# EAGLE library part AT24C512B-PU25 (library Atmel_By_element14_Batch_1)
Two-wire Serial EEPROM
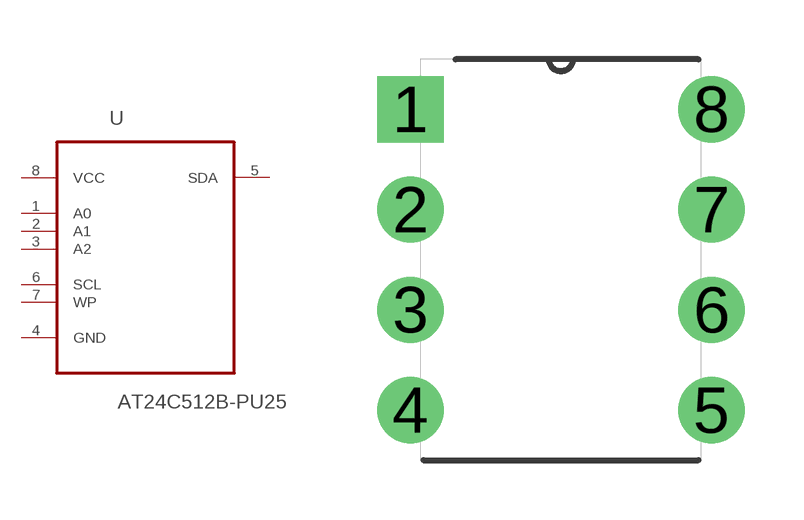
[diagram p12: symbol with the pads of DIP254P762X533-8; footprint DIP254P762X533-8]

Designator prefix U

## AT24C512B-PU25 (MPN: AT24C512B-PU25; OC_FARNELL: 1362655; OC_NEWARK: -; PACKAGE: PDIP-8; SUPPLIER: Atmel)  [DIP254P762X533-8]
1  A0  in
2  A1  in
3  A2  in
4  GND  pas
5  SDA
6  SCL  in
7  WP  pas
8  VCC  pwr

## Footprint DIP254P762X533-8 (pad centres in mm)
drill 1.118 square: 1 -7.62,7.62
drill 1.118: 2 -7.62,5.08; 3 -7.62,2.54; 4 -7.62,0; 5 0,0; 6 0,2.54; 7 0,5.08; 8 0,7.62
